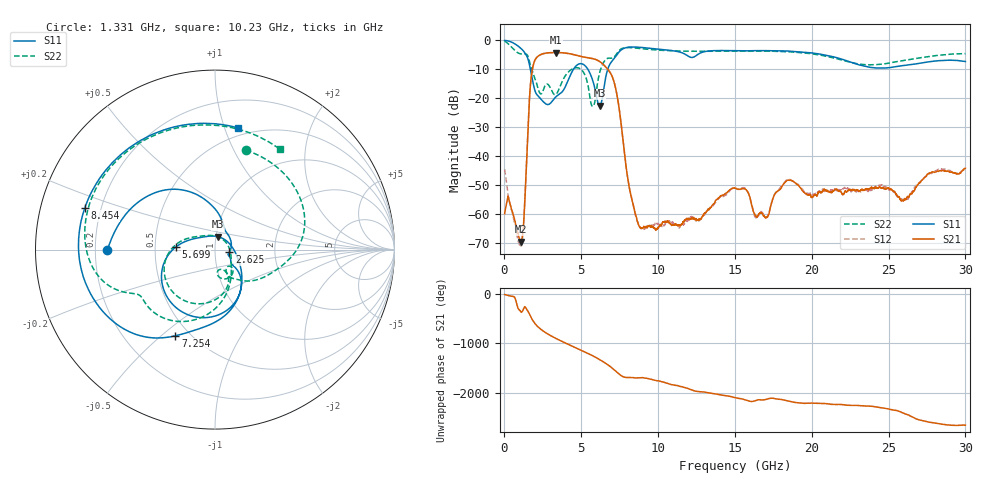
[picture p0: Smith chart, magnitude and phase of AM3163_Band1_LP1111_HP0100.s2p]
!Agilent Technologies,E8364B,MY43040894,A.07.50.67
!Agilent E8364B: A.07.50.67
!Date: Thursday, August 20, 2020 11:58:10
!Correction: S11(Full 2 Port(1,2))
!S21(Full 2 Port(1,2))
!S12(Full 2 Port(1,2))
!S22(Full 2 Port(1,2))
!S2P File: Measurements: S11, S21, S12, S22:
# Hz S  dB  R 50
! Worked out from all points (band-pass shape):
!   3201 points, 10 MHz to 30 GHz, reference 50 ohm
!   highest |S21| = -4.27 dB at 3.346 GHz (marker M1); lowest = -69.6 dB at 1.06 GHz (marker M2)
!   |S21| within 3 dB of the highest: 1.953 GHz to 6.163 GHz (4.21 GHz wide, 104 % of centre)
!   lowest |S11| = -22.6 dB at 6.186 GHz (marker M3), VSWR 1.16, Z = 51.3 + j7.38 ohm
!   |S11| at or under -10 dB: 1.683 GHz to 4.5 GHz (2.817 GHz wide, 91.1 % of centre); 5.422 GHz to 6.726 GHz (1.304 GHz wide, 21.5 % of centre)
!   |S22| runs from -22.9 to -0.4 dB; largest |S21 - S12| = 0.006
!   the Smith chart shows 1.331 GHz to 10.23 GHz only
!   S11 on the Smith chart (normalised r, x): 1.331 GHz: 0.25, -0.00; 2.625 GHz: 1.17, -0.03; 5.699 GHz: 0.64, +0.02; 7.254 GHz: 0.42, -0.56; 8.454 GHz: 0.14, +0.15; 10.23 GHz: 0.43, +1.12
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1e7  -0.10 -8.3  -60.00 -15.0  -44.60 76.9  -0.39 -15.2
4.504781e8  -0.65 -56.1  -58.41 -48.6  -58.29 -50.9  -2.33 -95.2
1.05965e9  -2.80 -136.0  -69.64 1.2  -70.78 40.9  -4.73 138.0
1.331434e9  -4.44 -179.6  -55.03 97.3  -54.81 149.4  -4.73 72.8
1.790656e9  -12.88 90.0  -10.97 -150.6  -10.98 -150.7  -10.25 -30.8
2.128044e9  -18.93 53.7  -5.82 68.4  -5.83 68.4  -15.63 -62.3
2.624753e9  -21.77 -9.7  -4.54 -54.9  -4.55 -54.9  -15.87 -51.7
3.346388e9  -19.59 -33.5  -4.27 178.1  -4.28 178.1  -18.76 -72.7
3.993047e9  -15.73 -42.1  -4.47 80.5  -4.50 80.5  -12.06 -79.9
5.014581e9  -8.14 -119.4  -5.67 -64.6  -5.66 -64.3  -10.24 -157.1
5.698728e9  -13.20 176.2  -6.33 -165.6  -6.30 -165.6  -22.77 74.1
6.186066e9  -22.64 75.8  -7.35 110.9  -7.38 110.7  -11.43 -78.3
7.254459e9  -5.54 -114.7  -17.08 -130.0  -17.07 -129.3  -5.09 -154.8
8.454059e9  -2.36 162.2  -58.61 100.0  -58.78 101.4  -2.68 132.4
1.000979e10  -3.11 88.3  -64.63 39.7  -63.46 41.5  -3.45 65.6
1.022534e10  -3.23 79.1  -63.95 22.2  -64.22 30.5  -3.53 57.3
1.5005e10  -3.59 -71.9  -51.21 58.4  -51.16 60.9  -3.79 -92.4
1.641078e10  -3.62 -105.9  -61.08 6.5  -61.55 9.6  -3.79 -126.8
2.000958e10  -4.40 162.7  -54.42 -49.9  -53.19 -58.0  -4.71 135.7
2.27368e10  -7.96 60.4  -51.74 -98.0  -51.88 -98.7  -7.92 20.9
2.500479e10  -9.52 -63.0  -51.10 -169.6  -51.69 -170.5  -7.96 -93.1
3e10  -7.39 104.8  -44.30 -137.4  -45.10 -131.4  -4.65 100.7
